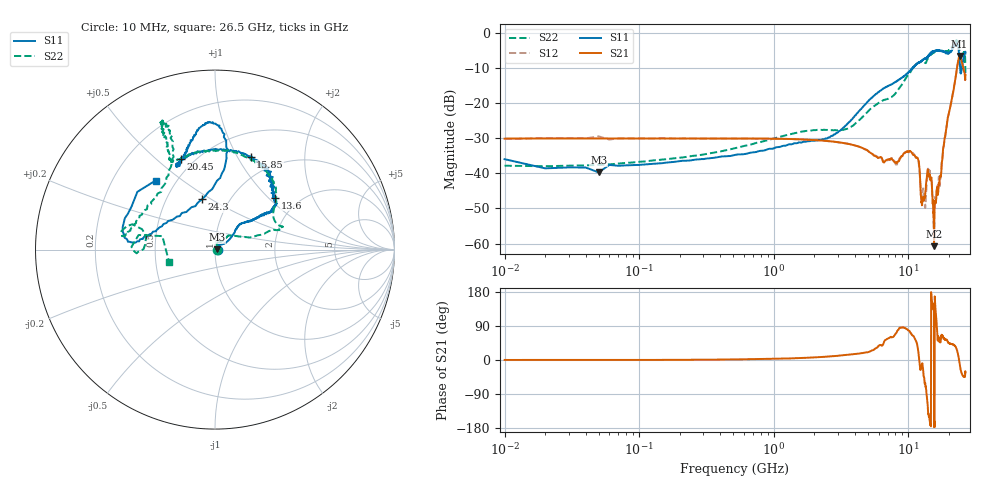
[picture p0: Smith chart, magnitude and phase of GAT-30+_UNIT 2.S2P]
!Created: 09-26-2013 at 09:17:58
!Mini-Circuits
!S2P DATA File Format
!Type: FIXED ATTENUATOR
!MODEL: GAT-30+
!S/N: Unit 2
!PIN OUT: PORT 1 - PIN 1, PORT 2 - PIN 3, GROUND - PIN 2,4
!TEST CONDITIONS: Z:50 OHM SYSTEM, INPUT POWER = -10dBm
!AP#: 130905
!PROD RUN: QM1142005 DATE CODE: 1142 WAFER/LOT#: WH461P005,AP130905
!REMARK: UNITS MOUNTED ON TB-154 D/C 1225. PORT EXTENSION HAS BEEN DONE.
!TESTED ON: NETWORK ANALYZER MODEL AG N5242A S/N 71932 CAL DUE DATE 3/15/14
# MHZ S DB R 50
! Frequency  S11 dB  S11 DEG  S21 dB  S21 DEG  S12 dB  S12 DEG  S22 dB  S22 DEG
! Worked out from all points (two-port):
!   930 points, 10 MHz to 26.5 GHz, reference 50 ohm
!   highest |S21| = -6.63 dB at 24 GHz (marker M1); lowest = -60.8 dB at 15.5 GHz (marker M2)
!   |S21| within 3 dB of the highest: 23.04 GHz to 25.44 GHz (2.409 GHz wide, 9.94 % of centre)
!   lowest |S11| = -39.8 dB at 50 MHz (marker M3), VSWR 1.02, Z = 51 + j0.235 ohm
!   |S11| at or under -10 dB: start of sweep to 10.7 GHz; 10.72654 GHz to 10.76225 GHz (35.72 MHz wide, 0.332 % of centre); 24.21 GHz to 24.93 GHz (719.5 MHz wide, 2.93 % of centre)
!   |S22| runs from -38.0 to -2.2 dB; largest |S21 - S12| = 0.0039
!   S11 on the Smith chart (normalised r, x): 10 MHz: 1.03, -0.01; 13.6 GHz: 1.53, +1.10; 15.85 GHz: 0.76, +1.14; 20.45 GHz: 0.43, +0.60; 24.3 GHz: 0.75, +0.46; 26.5 GHz: 0.39, +0.40
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10  -35.99 -9.2  -30.14 0.2  -30.23 7.2  -37.85 -11.3
40  -38.36 4.9  -30.07 0.1  -30.08 0.4  -37.77 7.4
50  -39.75 13.0  -30.06 0.1  -29.48 -3.9  -37.60 10.0
140  -37.17 19.7  -30.07 0.2  -30.05 0.2  -36.21 24.5
520  -34.75 40.1  -30.09 1.6  -30.09 1.4  -32.84 51.0
1920  -30.71 61.5  -30.50 6.6  -30.50 6.7  -27.78 86.5
3500  -26.02 36.0  -31.56 13.5  -31.57 13.7  -27.36 66.8
7150  -15.04 45.5  -36.09 57.6  -36.11 58.0  -18.68 42.5
10700  -9.97 36.2  -34.46 65.2  -34.11 66.3  -10.30 18.4
11850  -8.48 34.5  -36.16 22.1  -36.58 21.1  -8.55 17.3
12550  -8.07 35.2  -47.96 -13.8  -45.63 -3.8  -8.08 18.7
13250  -7.34 38.0  -46.95 -62.5  -49.46 -90.8  -8.50 22.0
13600  -7.07 40.8  -42.27 -86.7  -44.31 -77.9  -8.29 32.5
14550  -6.25 51.9  -41.90 -169.2  -41.06 -178.4  -6.42 45.2
15500  -5.19 64.2  -60.76 -176.7  -60.66 140.8  -5.56 58.4
15850  -5.11 69.1  -48.53 138.2  -46.82 143.0  -5.45 65.1
20450  -5.38 110.7  -21.14 42.7  -20.98 42.3  -4.75 115.6
22850  -3.02 91.7  -10.57 28.3  -10.56 28.2  -2.27 113.2
24000  -7.94 85.8  -6.63 -9.4  -6.63 -9.6  -5.50 117.2
24300  -10.77 104.5  -6.81 -21.0  -6.82 -21.0  -6.76 127.6
25850  -6.72 175.0  -10.87 -44.6  -10.94 -44.5  -5.50 168.7
26500  -5.89 130.7  -12.00 -33.2  -12.00 -33.5  -11.54 -165.4
